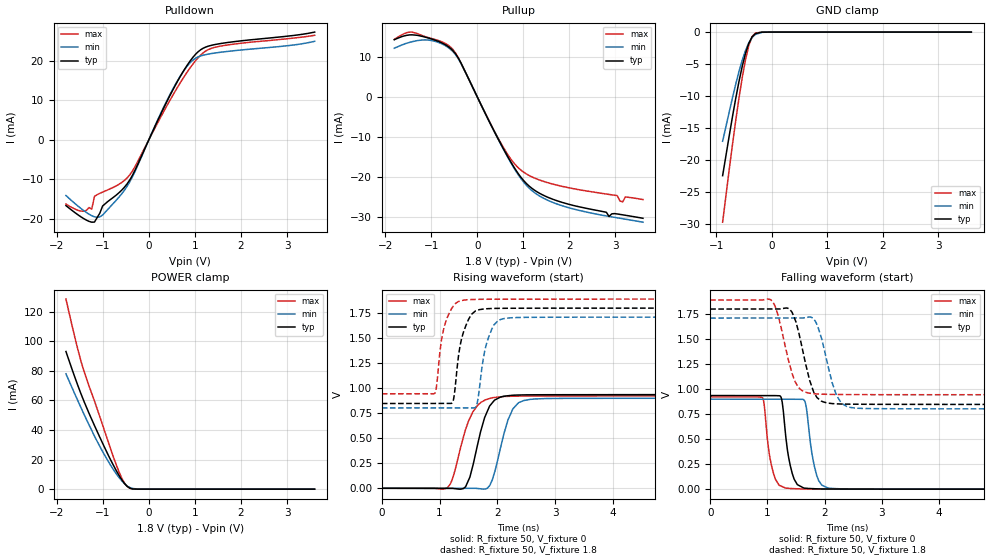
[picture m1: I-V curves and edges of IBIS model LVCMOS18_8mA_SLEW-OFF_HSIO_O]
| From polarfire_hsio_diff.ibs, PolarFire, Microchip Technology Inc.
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|   Model LVCMOS18_8mA_SLEW-OFF_HSIO_O
[Model]   LVCMOS18_8mA_SLEW-OFF_HSIO_O
Model_type   Output
Polarity   Non-Inverting
Enable   Active-High
Vmeas =   0.9
Cref =   5p
Rref =   1M
|   typ   min   max
C_comp_pullup   1.335e-12   1.335e-12   1.380e-12
C_comp_pulldown  1.335e-12   1.335e-12   1.380e-12
[Temperature Range]  25C   100C   -40C
[Voltage Range]  1.8   1.71   1.89
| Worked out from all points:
|   slope of the pulldown table from 0 to 0.27 V, typ, clamps not added: 40 ohm
|   slope of the pullup table from 0 to 0.27 V, typ, clamps not added: 42.5 ohm
|   GND clamp passes 1 mA (typ) near -0.37 V on its own axis
|   POWER clamp passes 1 mA (typ) near -0.43 V on its own axis
|   rising waveform, R_fixture 50, V_fixture 0: 20-80 % time 253ps typ, 250ps min, 287ps max; typ from 0 V to 0.936 V
|   rising waveform, R_fixture 50, V_fixture 1.8: 20-80 % time 170ps typ, 175ps min, 163ps max; typ from 0.847 V to 1.8 V
|   falling waveform, R_fixture 50, V_fixture 0: 20-80 % time 137ps typ, 141ps min, 132ps max; typ from 0.936 V to 0 V
|   falling waveform, R_fixture 50, V_fixture 1.8: 20-80 % time 241ps typ, 245ps min, 243ps max; typ from 1.8 V to 0.847 V
[GND Clamp]
| Voltage   I(typ)   I(min)   I(max)
-885.9mV  -22.44mA   -17.06mA   -29.71mA
-708.7mV  -13.24mA   -10.28mA   -17.6mA
-649.7mV  -10.37mA   -8.138mA   -13.83mA
-590.6mV  -7.705mA   -6.148mA   -10.3mA
-531.6mV  -5.322mA   -4.371mA   -7.074mA
-472.5mV  -3.308mA   -2.865mA   -4.286mA
-413.4mV  -1.757mA   -1.684mA   -2.101mA
-354.4mV  -739.5uA   -855.1uA   -713.7uA
-295.3mV  -232.3uA   -363.2uA   -148.3uA
-177.2mV  -12.01uA   -39.02uA   -3.177uA
-59.06mV  -489.8nA   -2.616uA   -234.3nA
3.6V      0A         0A         0A
[POWER Clamp]
| Voltage   I(typ)   I(min)   I(max)
-1.8V     93.11mA    78.02mA    128.6mA
-1.595V   74.64mA    63.48mA    101.1mA
-1.477V   64.73mA    55.33mA    86.9mA
-1.417V   60.07mA    51.32mA    80.62mA
-1.063V   35.01mA    28.82mA    48.84mA
-885.9mV  23.32mA    19.01mA    32.31mA
-708.7mV  12.62mA    10.48mA    16.53mA
-590.6mV  6.476mA    5.751mA    7.626mA
-472.5mV  1.932mA    2.149mA    1.873mA
-354.4mV  154uA      469.9uA    209.6uA
-236.2mV  4.969uA    79.11uA    56.46uA
3.6V      0A         0A         0A
[Pullup]
| Voltage   I(typ)   I(min)   I(max)
-1.8V     14.21mA    12.09mA    14.28mA
-1.417V   15.43mA    13.71mA    16.11mA
-945mV    14.22mA    13.9mA     14.37mA
-531.6mV  11.54mA    11.3mA     11.83mA
618.8mV   -14.01mA   -14.14mA   -13.59mA
900mV     -19.31mA   -19.59mA   -17.8mA
1.238V    -23.25mA   -23.85mA   -20.24mA
1.859V    -26.39mA   -27.23mA   -22.38mA
2.863V    -29.84mA   -29.83mA   -24.36mA
3.158V    -29.44mA   -30.41mA   -26.23mA
3.217V    -29.55mA   -30.53mA   -24.99mA
3.6V      -30.3mA    -31.28mA   -25.63mA
[Pulldown]
| Voltage   I(typ)   I(min)   I(max)
-1.8V     -16.63mA   -14.08mA   -16.23mA
-1.477V   -19.45mA   -17.33mA   -18.01mA
-1.24V    -20.82mA   -19.18mA   -17.54mA
-1.181V   -20.79mA   -19.46mA   -14.31mA
-1.004V   -16.72mA   -19.01mA   -13.21mA
-649.7mV  -13.39mA   -14.5mA    -11.25mA
-413.4mV  -10.13mA   -10.59mA   -8.855mA
562.5mV   13.49mA    13.7mA     12.08mA
843.8mV   19.02mA    18.77mA    17.3mA
1.125V    22.73mA    21.17mA    21.39mA
1.575V    24.33mA    22.13mA    23.69mA
3.6V      27.19mA    24.86mA    26.38mA
[Ramp]
dV/dt_r   0.561316/0.252913n  0.539654/0.25025n  0.553599/0.287206n
dV/dt_f   0.571987/0.241065n  0.54457/0.245252n  0.567798/0.2427n
R_load = 50
[Rising Waveform]
R_fixture = 50
V_fixture = 0
V_fixture_min = 0
V_fixture_max = 0
| Time   V(typ)   V(min)   V(max)
0s        2.497uV    2.678uV    4.909uV
1.139ns   -703.8uV   -486.2uV   7.035mV
1.249ns   -2.44mV    -533.4uV   143.9mV
1.413ns   -2.078mV   -603.8uV   513.4mV
1.577ns   230.1mV    -674.2uV   765.2mV
1.779ns   706.1mV    -7.32mV    878.9mV
1.914ns   855.2mV    87.42mV    904.6mV
2.269ns   929.4mV    793.9mV    919.6mV
2.563ns   933.5mV    887.6mV    921.3mV
10ns      935.5mV    899.4mV    922.7mV
[Rising Waveform]
R_fixture = 50
V_fixture = 1.8
V_fixture_min = 1.71
V_fixture_max = 1.89
| Time   V(typ)   V(min)   V(max)
0s        846.7mV    802.3mV    943.7mV
915ps     847.4mV    802.8mV    948.4mV
1.048ns   847.5mV    802.9mV    1.532V
1.212ns   850.2mV    803mV      1.8V
1.356ns   1.43V      803.1mV    1.87V
1.414ns   1.561V     803.1mV    1.879V
1.639ns   1.776V     826.7mV    1.887V
1.822ns   1.793V     1.465V     1.888V
2.085ns   1.797V     1.692V     1.889V
10ns      1.8V       1.71V      1.89V
[Falling Waveform]
R_fixture = 50
V_fixture = 0
V_fixture_min = 0
V_fixture_max = 0
| Time   V(typ)   V(min)   V(max)
0s        935.6mV    899.5mV    922.7mV
914ps     935.1mV    898.9mV    913.7mV
1.076ns   935mV      898.8mV    225.1mV
1.239ns   917.7mV    898.7mV    30.9mV
1.318ns   543.6mV    898.7mV    10.88mV
1.467ns   100.7mV    898.6mV    5.176mV
1.651ns   10.29mV    881.4mV    2.226mV
1.863ns   3.53mV     135.4mV    1.454mV
2.063ns   1.761mV    10.56mV    1.059mV
10ns      4.439uV    3.97uV     4.931uV
[Falling Waveform]
R_fixture = 50
V_fixture = 1.8
V_fixture_min = 1.71
V_fixture_max = 1.89
| Time   V(typ)   V(min)   V(max)
0s        1.8V       1.71V      1.89V
1.06ns    1.801V     1.711V     1.891V
1.184ns   1.801V     1.711V     1.744V
1.392ns   1.796V     1.711V     1.239V
1.531ns   1.603V     1.711V     1.026V
1.751ns   1.067V     1.72V      958mV
1.875ns   911.4mV    1.637V     951.1mV
2.208ns   852.6mV    936.9mV    946.3mV
2.462ns   849.4mV    815.6mV    945mV
10ns      846.7mV    802.3mV    943.6mV
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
